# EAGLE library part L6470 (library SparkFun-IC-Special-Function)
3A RMS/7A peak bipolar stepper motor driver with SPI control and step input in HTSSOP-28 package. IC-10648
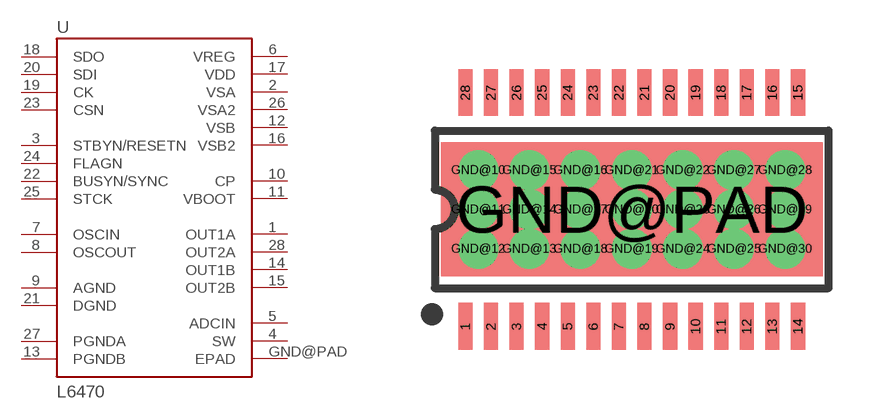
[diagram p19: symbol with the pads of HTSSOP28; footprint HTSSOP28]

Designator prefix U

## L6470 (PROD_ID: IC-10648)  [HTSSOP28]
1  OUT1A
2  VSA
3  STBYN/RESETN
4  SW
5  ADCIN
6  VREG
7  OSCIN
8  OSCOUT
9  AGND
10  CP
11  VBOOT
12  VSB
13  PGNDB
14  OUT1B
15  OUT2B
16  VSB2
17  VDD
18  SDO
19  CK
20  SDI
21  DGND
22  BUSYN/SYNC
23  CSN
24  FLAGN
25  STCK
26  VSA2
27  PGNDA
28  OUT2A
GND@PAD  EPAD

## Footprint HTSSOP28 (pad centres in mm)
smd 0.36 x 1.19: 1 -4.225,-2.97; 2 -3.575,-2.97; 3 -2.925,-2.97; 4 -2.275,-2.97; 5 -1.625,-2.97; 6 -0.975,-2.97; 7 -0.325,-2.97; 8 0.325,-2.97; 9 0.975,-2.97; 10 1.625,-2.97; 11 2.275,-2.97; 12 2.925,-2.97; 13 3.575,-2.97; 14 4.225,-2.97; 15 4.225,2.97; 16 3.575,2.97; 17 2.925,2.97; 18 2.275,2.97; 19 1.625,2.97; 20 0.975,2.97; 21 0.325,2.97; 22 -0.325,2.97; 23 -0.975,2.97; 24 -1.625,2.97; 25 -2.275,2.97; 26 -2.925,2.97; 27 -3.575,2.97; 28 -4.225,2.97
drill 0.508: GND@10 -3.9,1; GND@11 -3.9,0; GND@12 -3.9,-1; GND@13 -2.6,-1; GND@14 -2.6,0; GND@15 -2.6,1; GND@16 -1.3,1; GND@17 -1.3,0; GND@18 -1.3,-1; GND@19 0,-1; GND@20 0,0; GND@21 0,1; GND@22 1.3,1; GND@23 1.3,0; GND@24 1.3,-1; GND@25 2.6,-1; GND@26 2.6,0; GND@27 2.6,1; GND@28 3.9,1; GND@29 3.9,0; GND@30 3.9,-1
smd 9.7 x 3.4: GND@PAD 0,0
